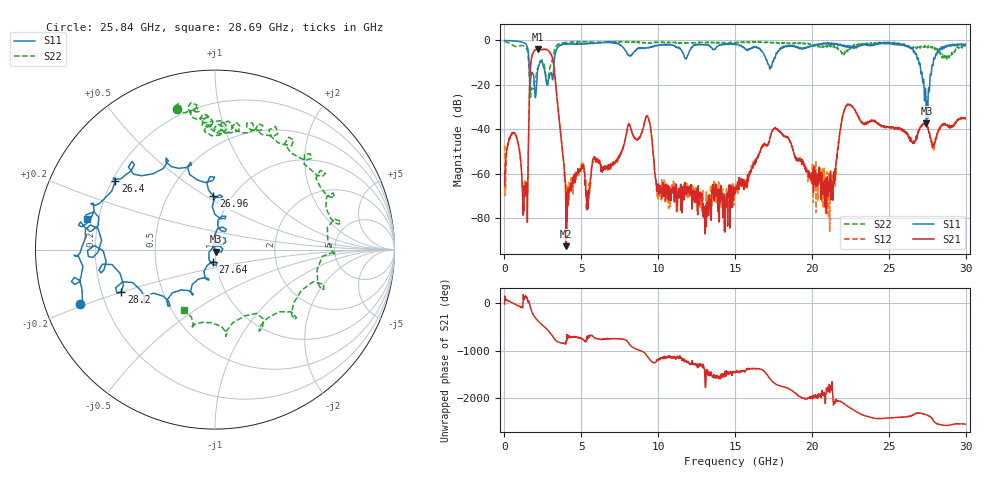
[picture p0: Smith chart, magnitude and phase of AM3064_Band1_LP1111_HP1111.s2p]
# Hz S DB R 50.0
!freq dBS11 angS11 dBS21 angS21 dBS12 angS12 dBS22 angS22
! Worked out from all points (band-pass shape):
!   1600 points, 10 MHz to 29.98 GHz, reference 50 ohm
!   highest |S21| = -3.97 dB at 2.203 GHz (marker M1); lowest = -92.5 dB at 4.021 GHz (marker M2)
!   |S21| within 3 dB of the highest: 1.788 GHz to 3.076 GHz (1.288 GHz wide, 52.9 % of centre)
!   lowest |S11| = -37.4 dB at 27.45 GHz (marker M3), VSWR 1.03, Z = 50.7 - j1.16 ohm
!   |S11| at or under -10 dB: 1.6 GHz to 2.307 GHz (707.4 MHz wide, 36.2 % of centre); 2.466 GHz to 3.226 GHz (759.7 MHz wide, 26.7 % of centre); 26.95 GHz to 27.89 GHz (938.5 MHz wide, 3.42 % of centre)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
!   |S22| runs from -25.5 to -0.2 dB; largest |S21 - S12| = 0.011
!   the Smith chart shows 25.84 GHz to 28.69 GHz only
!   S11 on the Smith chart (normalised r, x): 25.84 GHz: 0.11, -0.19; 26.4 GHz: 0.21, +0.30; 26.96 GHz: 0.82, +0.54; 27.64 GHz: 0.96, -0.13; 28.2 GHz: 0.28, -0.20; 28.69 GHz: 0.16, +0.12
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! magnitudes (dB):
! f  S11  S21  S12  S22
! 10 MHz  0.0  -65.4  -47.2  -0.2
! 666 MHz  -0.3  -41.8  -42.0  -2.6
! 1.36 GHz  -1.5  -65.3  -70.2  -2.7
! 1.753 GHz  -15.1  -8.2  -8.2  -21.6
! 2.203 GHz  -12.0  -4.0  -4.0  -11.4
! 3.14 GHz  -17.7  -8.5  -8.4  -8.0
! 4.021 GHz  -1.7  -92.5  -73.2  -1.0
! 5.015 GHz  -1.6  -57.7  -57.8  -0.5
! 9.288 GHz  -3.4  -34.0  -34.2  -1.4
! 10 GHz  -2.2  -64.5  -71.3  -0.9
! 15 GHz  -1.8  -67.3  -66.6  -1.1
! 17.59 GHz  -7.9  -39.6  -39.2  -0.9
! 19.99 GHz  -2.7  -59.6  -60.1  -1.7
! 25 GHz  -1.0  -38.8  -39.1  -1.1
! 25.84 GHz  -1.8  -39.9  -40.1  -1.8
! 26.4 GHz  -3.4  -44.7  -44.0  -3.1
! 26.96 GHz  -10.5  -40.5  -40.2  -3.1
! 27.45 GHz  -37.4  -38.8  -38.8  -2.5
! 27.64 GHz  -23.1  -41.7  -41.4  -3.1
! 28.2 GHz  -4.8  -41.2  -40.6  -4.8
! 28.69 GHz  -2.7  -37.9  -37.8  -8.4
! 29.98 GHz  -1.7  -35.2  -35.0  -2.9
